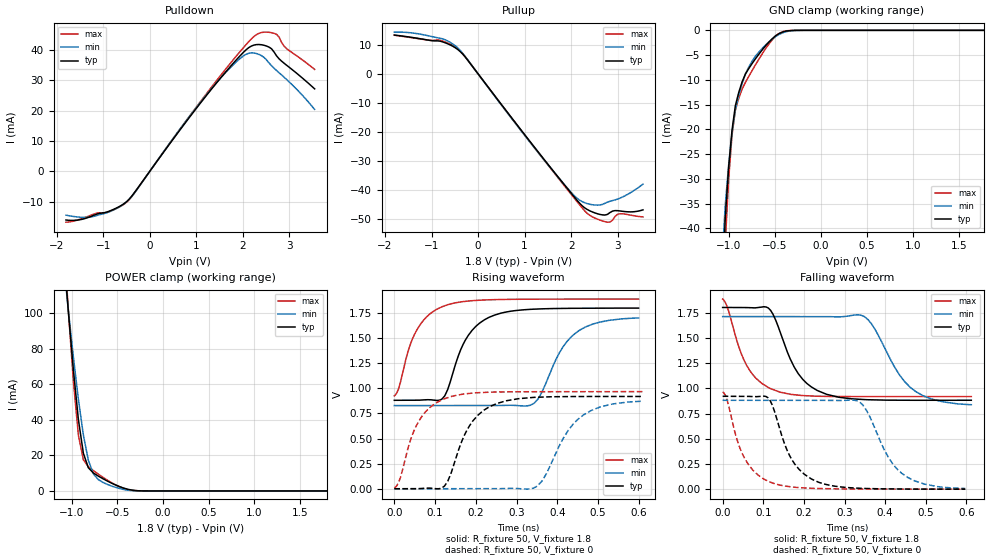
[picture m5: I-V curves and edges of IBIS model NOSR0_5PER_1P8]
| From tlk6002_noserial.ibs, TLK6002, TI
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[Model]   NOSR0_5PER_1P8
Model_type   3-state
Polarity   Non-Inverting
Enable   Active-Low
Cref =  15.0000pF
Rref =  100.0000M
Vref =  0V
Vmeas =  0.9
C_comp   1.885425p   1.715283p   2.176444p
[Temperature Range]   25   125   -40
[Voltage Range]   1.8   1.71   1.89
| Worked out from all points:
|   slope of the pulldown table from 0 to 0.27 V, typ, clamps not added: 47.1 ohm
|   slope of the pullup table from 0 to 0.27 V, typ, clamps not added: 47.4 ohm
|   GND clamp passes 1 mA (typ) near -0.48 V on its own axis
|   POWER clamp passes 1 mA (typ) near -0.39 V on its own axis
|   rising waveform, R_fixture 50, V_fixture 1.8: 20-80 % time 62.2ps typ, 70.9ps min, 57.1ps max; typ from 0.881 V to 1.8 V
|   rising waveform, R_fixture 50, V_fixture 0: 20-80 % time 64.3ps typ, 76.4ps min, 57.9ps max; typ from 0 V to 0.919 V
|   falling waveform, R_fixture 50, V_fixture 1.8: 20-80 % time 66.6ps typ, 79.4ps min, 59.4ps max; typ from 1.8 V to 0.882 V
|   falling waveform, R_fixture 50, V_fixture 0: 20-80 % time 60.9ps typ, 70.2ps min, 55.2ps max; typ from 0.921 V to 0.002 V
[POWER_clamp]
-1.8V     644.6mA    525mA      776.9mA
-1.055V   111.8mA    110.1mA    115.1mA
-1.036V   100.1mA    100.9mA    100.7mA
-981.8mV  67.73mA    75.06mA    61.45mA
-927.3mV  40.06mA    51.42mA    31.31mA
-872.7mV  21.16mA    31.46mA    17.46mA
-818.2mV  13.02mA    17.22mA    13.64mA
-763.6mV  10.12mA    9.635mA    11.46mA
-654.5mV  6.765mA    4.687mA    7.549mA
-436.4mV  1.678mA    857.7uA    1.497mA
-272.7mV  101.6uA    39.45uA    61.06uA
1.8V      90.02nA    124.6nA    271nA
[Pulldown]
-1.8V     -16mA      -14.39mA   -16.72mA
-1.2V     -14.43mA   -14.79mA   -14.05mA
-872.7mV  -13.11mA   -13.32mA   -13.24mA
-490.9mV  -9.876mA   -9.958mA   -10.07mA
1.2V      24.63mA    24.88mA    25.17mA
1.691V    33.76mA    33.5mA     34.78mA
2.073V    40.05mA    38.56mA    41.76mA
2.4V      41.7mA     38.12mA    45.7mA
2.673V    39.31mA    33.97mA    45.46mA
2.782V    37.05mA    32.46mA    44.2mA
2.945V    34.92mA    30.22mA    40.39mA
3.545V    27.17mA    20.41mA    33.58mA
[Pullup]
-1.8V     13.31mA    14.32mA    13.24mA
-763.6mV  10.98mA    12.02mA    11.23mA
-436.4mV  8.351mA    8.912mA    8.593mA
-272.7mV  5.714mA    5.884mA    5.754mA
1.364V    -28.29mA   -28.5mA    -28.48mA
2.182V    -44.46mA   -43.42mA   -45.01mA
2.4V      -47.09mA   -44.84mA   -48.63mA
2.618V    -48.34mA   -45.11mA   -50.27mA
2.782V    -48.32mA   -44.12mA   -51.01mA
2.891V    -47.2mA    -43.59mA   -50.31mA
3.055V    -47.16mA   -42.72mA   -48.1mA
3.545V    -46.77mA   -37.91mA   -49.18mA
[GND_clamp]
-1.8V     -566.4mA   -409.5mA   -760.6mA
-1.073V   -54mA      -46.59mA   -65.56mA
-1.036V   -37.78mA   -35.22mA   -42.81mA
-1V       -27.67mA   -27.21mA   -30.08mA
-963.6mV  -20.15mA   -20.81mA   -21.17mA
-927.3mV  -15.22mA   -16.02mA   -16.11mA
-890.9mV  -12.56mA   -13.16mA   -13.75mA
-818.2mV  -8.811mA   -8.808mA   -10.5mA
-745.5mV  -6.683mA   -6.209mA   -8.111mA
-454.5mV  -667.9uA   -843.8uA   -644.4uA
-236.4mV  -5uA       -16.85uA   -2.331uA
1.764V    74.33nA    230.2nA    154.6nA
[Ramp]
dV/dt_f  0.4628854/52.39885p   0.4493348/64.94453p   0.4871601/46.54088p
dV/dt_r  0.4608683/50.50782p   0.4427082/61.55637p   0.4847/45.29979p
R_load = 50
[Rising Waveform]
R_fixture = 50
V_fixture = 1.8
V_fixture_min = 1.71
V_fixture_max = 1.89
0s        881.4mV    828.6mV    925.4mV
54ps      881.5mV    828.6mV    1.573V
116ps     891.9mV    828.6mV    1.812V
131ps     988.4mV    828.6mV    1.834V
174ps     1.479V     828.7mV    1.867V
232ps     1.707V     828mV      1.883V
342ps     1.789V     849.2mV    1.889V
404ps     1.796V     1.348V     1.89V
443ps     1.798V     1.546V     1.89V
599ps     1.8V       1.701V     1.89V
[Rising Waveform]
R_fixture = 50
V_fixture = 0
V_fixture_min = 0
V_fixture_max = 0
0s        9.876uV    1.221uV    7.64mV
15ps      13.55uV    1.21uV     110.8mV
59ps      879.3uV    1.178uV    665.9mV
119ps     14.86mV    -1.771uV   890.9mV
183ps     618.4mV    51.5uV     949.7mV
249ps     845.9mV    -295.8uV   963.9mV
350ps     911.7mV    24.44mV    966.8mV
425ps     918.7mV    572.1mV    967mV
463ps     919.3mV    732.9mV    967.1mV
610ps     919.5mV    872.7mV    967.6mV
[Falling Waveform]
R_fixture = 50
V_fixture = 1.8
V_fixture_min = 1.71
V_fixture_max = 1.89
0s        1.8V       1.71V      1.883V
13ps      1.8V       1.71V      1.786V
58ps      1.799V     1.71V      1.234V
115ps     1.784V     1.71V      1.002V
175ps     1.218V     1.71V      936.7mV
233ps     978.1mV    1.711V     921.4mV
349ps     887.6mV    1.709V     917.8mV
461ps     881.5mV    1.012V     917.9mV
512ps     881.5mV    896.2mV    917.8mV
612ps     881.7mV    837.5mV    917.8mV
[Falling Waveform]
R_fixture = 50
V_fixture = 0
V_fixture_min = 0
V_fixture_max = 0
0s        920.9mV    881.3mV    964.2mV
11ps      920.9mV    881.3mV    884.8mV
53ps      921mV      881.3mV    315mV
115ps     889.2mV    881.3mV    74.24mV
170ps     296mV      881.3mV    23.78mV
235ps     71.73mV    882mV      8.082mV
338ps     10.58mV    860.7mV    3.128mV
408ps     4.168mV    314.8mV    2.454mV
453ps     2.813mV    123.6mV    2.228mV
597ps     1.728mV    8.704mV    1.835mV
